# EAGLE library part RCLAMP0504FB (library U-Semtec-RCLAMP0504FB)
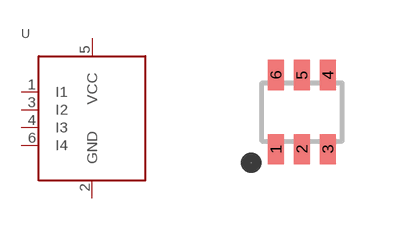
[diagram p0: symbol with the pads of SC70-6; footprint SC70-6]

Designator prefix U

## RCLAMP0504FB  [SC70-6]
1  I1
2  GND  sup
3  I2
4  I3
5  VCC  pwr
6  I4

## Footprint SC70-6 (pad centres in mm)
smd 0.4 x 0.75: 1 -0.65,-0.925; 2 0,-0.925; 3 0.65,-0.925; 4 0.65,0.925; 5 0,0.925; 6 -0.65,0.925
